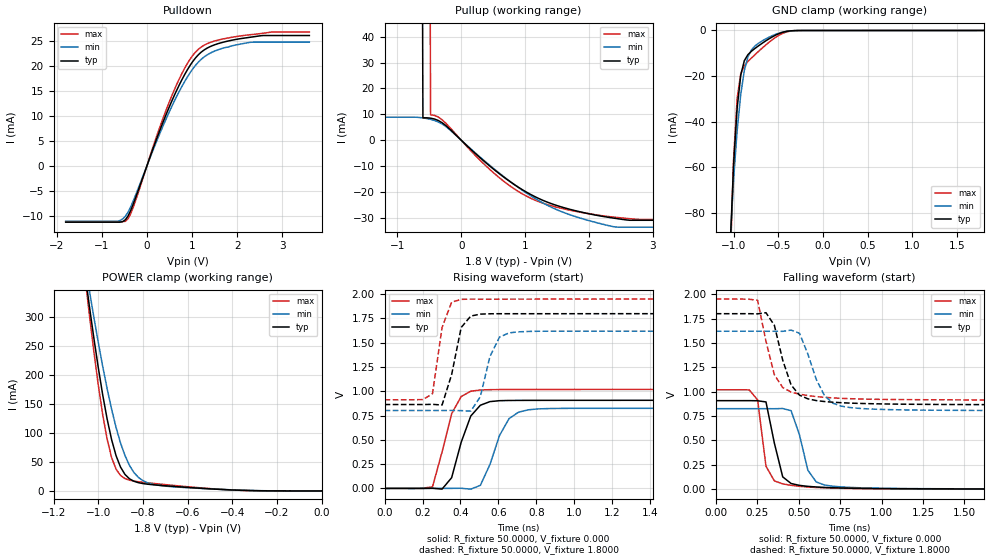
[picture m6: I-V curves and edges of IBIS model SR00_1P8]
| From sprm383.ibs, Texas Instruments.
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|   Model BHSTLDVG_SR00_1P8
[Model]   SR00_1P8
Model_type   I/O
Polarity   Non-Inverting
Enable   Active-Low
Vinl =   0.8000V
Vinh =   1.0000V
Vmeas =   0.9000V
Cref =   5.0000pF
Rref =  50.0000
Vref =   0.9000V
C_comp   1.2405pF   1.1811pF   1.2768pF
[Temperature Range]   25.0000   0.1250k   -40.0000
[Pullup Reference]   1.8000V   1.6200V   1.9500V
[Pulldown Reference]   0.000V   0.000V   0.000V
[POWER Clamp Reference]   1.8000V   1.6200V   1.9500V
[GND Clamp Reference]   0.000V   0.000V   0.000V
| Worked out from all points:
|   slope of the pulldown table from 0 to 0.27 V, typ, clamps not added: 40.2 ohm
|   slope of the pullup table from 0 to 0.27 V, typ, clamps not added: 43.4 ohm
|   GND clamp passes 1 mA (typ) near -0.47 V on its own axis
|   POWER clamp passes 1 mA (typ) near -0.35 V on its own axis
|   rising waveform, R_fixture 50.0000, V_fixture 0.000: 20-80 % time 87.5ps typ, 103ps min, 88ps max; typ from 0 V to 0.908 V
|   rising waveform, R_fixture 50.0000, V_fixture 1.8000: 20-80 % time 65.3ps typ, 72.6ps min, 56.3ps max; typ from 0.864 V to 1.8 V
|   falling waveform, R_fixture 50.0000, V_fixture 0.000: 20-80 % time 72.7ps typ, 83.6ps min, 53.7ps max; typ from 0.908 V to 0 V
|   falling waveform, R_fixture 50.0000, V_fixture 1.8000: 20-80 % time 99.8ps typ, 115ps min, 98.1ps max; typ from 1.8 V to 0.864 V
[Pulldown]
| voltage   I(typ)   I(min)   I(max)
-1.8V     -11.26mA   -11.09mA   -11.14mA
-600mV    -11.26mA   -10.94mA   NA
-480mV    -10.79mA   -10.1mA    -11.09mA
-420mV    -10.05mA   -9.293mA   -10.6mA
-300mV    -7.566mA   -6.939mA   -8.201mA
240mV     6mA        5.466mA    6.559mA
600mV     13.94mA    12.8mA     15.05mA
900mV     19.26mA    17.82mA    20.52mA
1.2V      22.71mA    21.27mA    23.73mA
1.62V     24.55mA    23.35mA    25.24mA
2.28V     25.7mA     24.68mA    26.21mA
3.6V      26.06mA    24.73mA    26.74mA
[Pullup]
| voltage   I(typ)   I(min)   I(max)
-1.8V     8.672A     8.909mA    9.806A
-600mV    8.672mA    8.62mA     NA
-540mV    8.657mA    8.383mA    NA
-480mV    8.52mA     8.062mA    9.806mA
-300mV    6.774mA    6.277mA    7.914mA
420mV     -9.432mA   -9.157mA   -10.69mA
960mV     -19.18mA   -19.4mA    -20.8mA
1.2V      -22.38mA   -23.16mA   -23.65mA
1.56V     -25.75mA   -27.53mA   -26.3mA
2.34V     -29.97mA   -33.23mA   -29.63mA
2.64V     -30.99mA   NA         -30.37mA
3.48V     -30.99mA   -33.66mA   -30.73mA
[GND_clamp]
| voltage   I(typ)   I(min)   I(max)
-1.8V     -3.609A    -2.85A     -4.282A
-1.04V    -96.53mA   -94.33mA   -105.1mA
-1V       -58.65mA   -65.31mA   -56.38mA
-960mV    -33.96mA   -43.86mA   -29.68mA
-920mV    -19.62mA   -28.07mA   -18.93mA
-880mV    -13.26mA   -17.54mA   -15.46mA
-840mV    -10.62mA   -11.58mA   -13.62mA
-800mV    -9.09mA    -8.506mA   -12.07mA
-680mV    -5.604mA   -4.576mA   -7.722mA
-480mV    -1.184mA   -1mA       -1.81mA
-320mV    -54.22uA   -73.53uA   -86.28uA
1.8V      123.7nA    73.42uA    85.3nA
[POWER_clamp]
| voltage   I(typ)   I(min)   I(max)
-1.8V     2.926A     2.488A     3.341A
-1.06V    376.9mA    393.7mA    372mA
-1.04V    319.5mA    346.2mA    305.1mA
-1.02V    264.7mA    300.3mA    241.8mA
-1V       213.2mA    256.4mA    183.4mA
-960mV    123.8mA    176.1mA    89.05mA
-940mV    88.38mA    140.7mA    57.5mA
-920mV    60.69mA    109.3mA    37.47mA
-880mV    28.35mA    60.73mA    21.23mA
-820mV    14.22mA    23.32mA    15.8mA
-740mV    10.13mA    10.22mA    12.43mA
0V        123.7nA    145.3nA    196.3nA
[Ramp]
| variable   typ   min   max
dV/dt_r   0.5449/87.1978p   0.4953/0.1021n   0.6119/87.0757p
dV/dt_f   0.5615/98.8268p   0.4900/0.1138n   0.6220/97.1326p
R_load = 50.0000
[Rising Waveform]
R_fixture = 50.0000
V_fixture = 0.000
V_fixture_min = 0.000
V_fixture_max = 0.000
| time   V(typ)   V(min)   V(max)
0s        49.37uV    69.14uV    51.62uV
252.5ps   2.44mV     73.19uV    16.02mV
303ps     -7.035mV   49.74uV    375.3mV
353.5ps   110.1mV    505.8uV    768.9mV
404ps     475.8mV    1.79mV     946.2mV
454.5ps   745.7mV    -7.672mV   1.001V
505.1ps   856.6mV    31.55mV    1.014V
656.6ps   905.7mV    719mV      1.018V
808.1ps   906.9mV    818.6mV    1.019V
5ns       908.1mV    825.6mV    1.02V
[Rising Waveform]
R_fixture = 50.0000
V_fixture = 1.8000
V_fixture_min = 1.6200
V_fixture_max = 1.9500
| time   V(typ)   V(min)   V(max)
0s        863.7mV    802.5mV    912.8mV
252.5ps   865.9mV    802.5mV    975mV
303ps     858.7mV    802.5mV    1.657V
353.5ps   1.172V     803.1mV    1.917V
404ps     1.658V     801.2mV    1.947V
505.1ps   1.795V     945.2mV    1.949V
555.6ps   1.798V     1.358V     1.949V
606.1ps   1.799V     1.559V     1.949V
707.1ps   1.799V     1.613V     1.949V
5ns       1.8V       1.62V      1.95V
[Falling Waveform]
R_fixture = 50.0000
V_fixture = 0.000
V_fixture_min = 0.000
V_fixture_max = 0.000
| time   V(typ)   V(min)   V(max)
0s        908.2mV    825.8mV    1.02V
202ps     908.2mV    825.8mV    1.018V
252.5ps   907mV      825.8mV    915.5mV
303ps     895mV      825.8mV    235.7mV
404ps     126.2mV    827.7mV    54.47mV
454.5ps   58.31mV    805mV      39.53mV
555.6ps   29.15mV    194mV      22.53mV
606.1ps   22.64mV    74.18mV    17.43mV
707.1ps   14.77mV    30.58mV    10.93mV
5ns       380uV      633.9uV    299.1uV
[Falling Waveform]
R_fixture = 50.0000
V_fixture = 1.8000
V_fixture_min = 1.6200
V_fixture_max = 1.9500
| time   V(typ)   V(min)   V(max)
0s        1.8V       1.62V      1.95V
252.5ps   1.798V     1.62V      1.937V
303ps     1.81V      1.62V      1.518V
353.5ps   1.681V     1.62V      1.174V
404ps     1.323V     1.619V     1.042V
505.1ps   964.4mV    1.599V     974.3mV
555.6ps   926.6mV    1.386V     960.2mV
656.6ps   898.8mV    957.3mV    942.1mV
858.6ps   880.2mV    829.7mV    925.7mV
5ns       864.2mV    803.3mV    913.3mV
